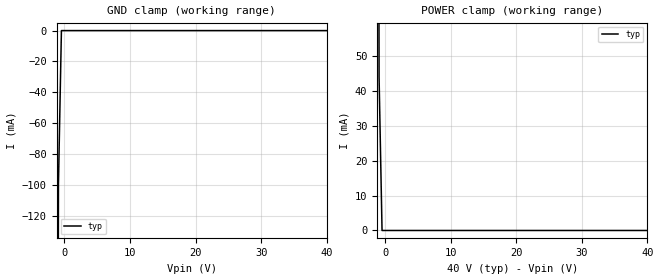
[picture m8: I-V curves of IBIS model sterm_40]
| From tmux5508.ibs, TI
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| sterm_40
[Model]   sterm_40
Model_type   Terminator
|   typ   min   max
C_comp   2.533030e-12   NA   NA
[Voltage Range]   40   NA   NA
[Temperature Range]   27   NA   NA
[Power Clamp Reference]   40   NA   NA
[GND Clamp Reference]   0   NA   NA
[GND Clamp]
|   Voltage   I(typ)   I(min)   I(max)
-5V       -13.02A    NA         NA
-1.364V   -1.178A    NA         NA
-909.1mV  -99.73mA   NA         NA
-454.5mV  -820.3nA   NA         NA
40V       660nA      NA         NA
[POWER Clamp]
|   Voltage   I(typ)   I(min)   I(max)
-5V       6.669A     NA         NA
-1.364V   578.8mA    NA         NA
-909.1mV  44.16mA    NA         NA
-454.5mV  672.1nA    NA         NA
40V       -4.292nA   NA         NA
